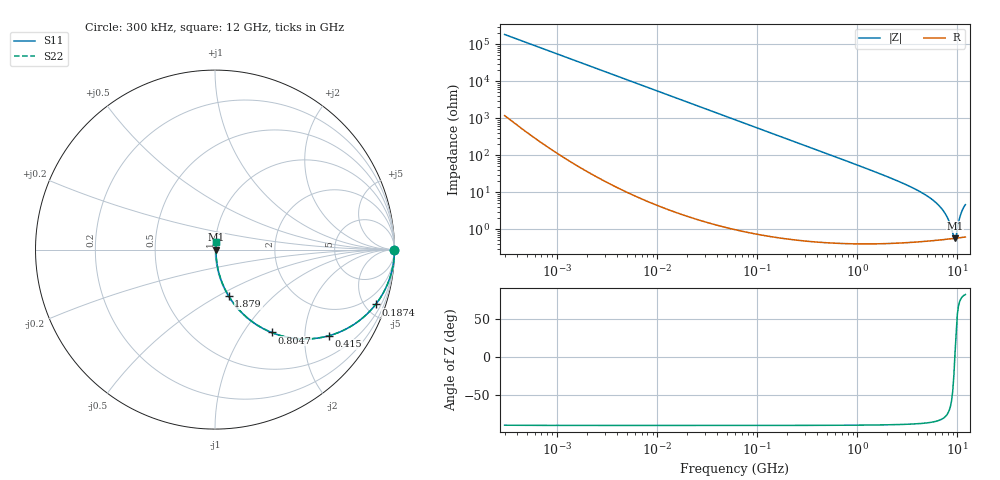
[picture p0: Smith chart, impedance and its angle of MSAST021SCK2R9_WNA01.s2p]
! MSAST021SCK2R9_WNA01  S-PARAMETER MODEL  ( General Type )
! Model Generated by TAIYO YUDEN Corporation (http://www.ty-top.com)
! Version 2.0
! TAIYO YUDEN Control No. 181101
! Copyright(c) 2015 TAIYO YUDEN CO.,LTD. All Rights Reserved.
! Product Description (link to TY-COMPAS)
! https://ds.yuden.co.jp/TYCOMPAS/or/detail?pn=MSAST021SCK2R9BWNA01&u=M
! Products Name : Multilayer Ceramic Capacitors
! Characteristics :
!  Capacitance : 2.9 pF , Rated Voltage : 25V , TCC : CK / C0K
!  Case Size : 0.25 x 0.125 / 0.0098 x 0.0049 [mm/inch] , Thickness : 0.125 / 0.0049 [mm/inch]
!  (Conditions: Temperature = 25 degC , DC Bias Current/Voltage = 0A / 0V)
! External Node Assignments :
!  1  o---| |---o  2
! GND o---------o GND
! Frequency Range : 0.3MHz  -  12000MHz  [ 401 STEP ]
# MHz S RI R 50
! Freq[MHz].  S11 Real  S11 Imag  S21 Real  S21 Imag  S12 Real  S12 Imag  S22 Real  S22 Imag
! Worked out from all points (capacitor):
!   401 points, 300 kHz to 12 GHz, reference 50 ohm
!   read as one part in series: C = 2.9 pF near 316.3 kHz
!   lowest |Z| = 572 mohm at 9.454 GHz (marker M1)
!   series resonance near 9.413 GHz, so ESL is about 99 pH
!   S11 on the Smith chart (normalised r, x): 300 kHz: open; 187.4 MHz: 1.01, -5.85; 415 MHz: 1.01, -2.64; 804.7 MHz: 1.01, -1.35; 1.879 GHz: 1.01, -0.56; 12 GHz: 1.01, +0.09
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0.3  1 -0.000547  3.81e-06 0.000547  3.81e-06 0.000547  1 -0.000547
1.769972  1 -0.00323  1.49e-05 0.00323  1.49e-05 0.00323  1 -0.00323
10.44266  0.9996 -0.019  0.000377 0.019  0.000377 0.019  0.9996 -0.019
60  0.9881 -0.108  0.0119 0.108  0.0119 0.108  0.9881 -0.108
187.4445  0.895 -0.3056  0.105 0.3056  0.105 0.3056  0.895 -0.3056
353.9943  0.705 -0.4545  0.295 0.4545  0.295 0.4545  0.705 -0.4545
414.98  0.6349 -0.4798  0.3651 0.4798  0.3651 0.4798  0.6349 -0.4798
804.7407  0.3153 -0.4616  0.6847 0.4616  0.6847 0.4616  0.3153 -0.4616
1229.528  0.1637 -0.3654  0.8363 0.3654  0.8363 0.3654  0.1637 -0.3654
1878.541  0.0762 -0.2581  0.9238 0.2581  0.9238 0.2581  0.0762 -0.2581
2088.533  0.0622 -0.2333  0.9378 0.2333  0.9378 0.2333  0.0622 -0.2333
4050.141  0.0164 -0.1081  0.9836 0.1081  0.9836 0.1081  0.0164 -0.1081
6026.253  0.0078 -0.053  0.9922 0.053  0.9922 0.053  0.0078 -0.053
7448.838  0.006 -0.0272  0.994 0.0272  0.994 0.0272  0.006 -0.0272
8064.993  0.00571 -0.0178  0.9943 0.0178  0.9943 0.0178  0.00571 -0.0178
8966.534  0.0056 -0.00554  0.9944 0.00554  0.9944 0.00554  0.0056 -0.00554
9207.246  0.00562 -0.00248  0.9944 0.00248  0.9944 0.00248  0.00562 -0.00248
9454.42  0.00566 0.000498  0.9943 -0.000498  0.9943 -0.000498  0.00566 0.000498
9968.853  0.00583 0.00851  0.9942 -0.00851  0.9942 -0.00851  0.00583 0.00851
10511.28  0.00623 0.0191  0.9938 -0.0191  0.9938 -0.0191  0.00623 0.0191
11083.22  0.00688 0.0302  0.9931 -0.0302  0.9931 -0.0302  0.00688 0.0302
12000  0.00818 0.0451  0.9918 -0.0451  0.9918 -0.0451  0.00818 0.0451
